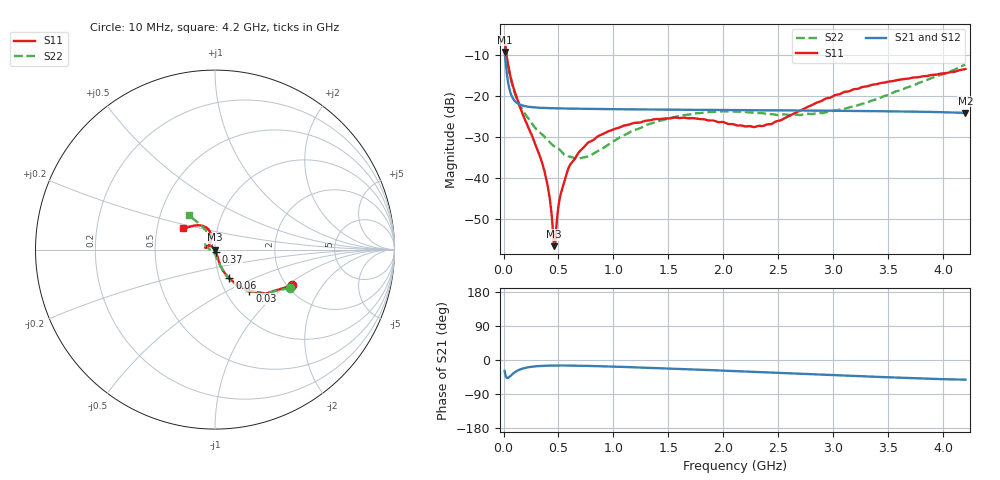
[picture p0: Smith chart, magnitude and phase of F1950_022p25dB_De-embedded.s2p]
! Integrated Device Technology
! Corporate Headquarters
! 6024 Silver Creek Valley Road
! San Jose, CA 95138  USA
! Phone:  1-408-284-8200
! Toll Free:  1-800-223-1366
! Webpage:  http://www.idt.com/
! Timing and RF Division
! 515 Groton Road, Suite 102
! Westford, MA 01886-6024
! Device:  F1950
! Description: 7-bit 0.25 dB Digital Step Attenuator
! Frequency:  150.0 -  4000.00 MHz
! Package:  4x4 mm Thin QFN Plastic Package: 24 pin
! Ports:  2 RF, 12 DC
!  Pin  1  = D0
!  Pin  2  = VDD
!  Pin  3  = Vmode
!  Pin  4  = GND
!  Pin  5  = RF1  =  Port 1
!  Pin  6  = GND
!  Pin  7  = GND
!  Pin  8  = GND
!  Pin  9  = GND
!  Pin 10  = GND
!  Pin 11  = GND
!  Pin 12  = GND
!  Pin 13  = GND
!  Pin 14  = RF2  =  Port 2
!  Pin 15  = GND
!  Pin 16  = LE
!  Pin 17  = CLK
!  Pin 18  = DATE
!  Pin 19  = D6
!  Pin 20  = D5
!  Pin 21  = D4
!  Pin 22  = D3
!  Pin 23  = D2
!  Pin 24  = D1
! State:  89
! Atten State:  22.25 dB
! Voltage:  +5.00 Volts
! Current:  Not Measured mA
! Data:  The device was measured on a the F195X evaluation board which has
!  individual transmission lines to the RF pins.  Data was collected
!  using a calibrated network analyzer.  The evaluation board was
!  de-embedded using a TRL calibration technique.
!  The reference plane is the edge of the package pin.
! Misc:  Board 2019
!  Action Tracker AT0250
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# GHz S dB R 50
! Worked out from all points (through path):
!   420 points, 10 MHz to 4.2 GHz, reference 50 ohm
!   highest |S21| = -9.31 dB at 10 MHz (marker M1); lowest = -24.1 dB at 4.2 GHz (marker M2)
!   group delay of S21, straight-line fit = 24.8 ps
!   lowest |S11| = -56.6 dB at 460 MHz (marker M3), VSWR 1.00, Z = 49.9 - j0.107 ohm
!   |S11| at or under -10 dB: 27.45 MHz to end of sweep
!   |S22| runs from -35.4 to -6.6 dB; largest |S21 - S12| = 0.00011
!   S11 on the Smith chart (normalised r, x): 10 MHz: 2.12, -1.09; 30 MHz: 1.29, -0.65; 60 MHz: 1.11, -0.37; 370 MHz: 1.01, -0.02; 4.2 GHz: 0.68, +0.17
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0.01  -6.52 -25.0  -9.31 -28.9  -9.31 -28.9  -6.61 -27.1
0.03  -10.49 -50.1  -14.54 -47.4  -14.54 -47.4  -10.80 -52.4
0.06  -14.94 -63.3  -18.95 -42.9  -18.95 -42.9  -15.12 -64.8
0.1  -18.82 -70.1  -21.16 -32.8  -21.16 -32.8  -19.17 -70.0
0.16  -23.48 -72.0  -22.24 -23.9  -22.24 -23.9  -22.86 -74.8
0.31  -33.26 -71.1  -22.87 -16.3  -22.87 -16.3  -28.42 -82.0
0.37  -38.06 -68.6  -22.95 -15.3  -22.95 -15.3  -29.87 -84.6
0.41  -43.20 -75.1  -22.99 -14.9  -22.99 -14.9  -31.01 -86.5
0.45  -52.95 -101.7  -23.02 -14.6  -23.02 -14.6  -32.05 -92.1
0.46  -56.58 -133.7  -23.03 -14.6  -23.03 -14.6  -32.25 -93.8
0.48  -52.00 155.4  -23.04 -14.5  -23.04 -14.5  -32.55 -96.7
0.52  -43.94 140.0  -23.06 -14.5  -23.06 -14.5  -33.35 -100.2
0.58  -38.41 135.0  -23.09 -14.6  -23.09 -14.6  -34.74 -112.7
0.71  -33.03 138.0  -23.14 -15.2  -23.14 -15.2  -35.09 -138.6
0.95  -28.70 146.4  -23.22 -17.0  -23.22 -17.0  -31.92 -176.3
1.41  -25.65 163.4  -23.34 -21.5  -23.35 -21.5  -26.13 160.8
1.73  -25.43 168.9  -23.40 -24.9  -23.40 -24.9  -24.30 152.4
2.11  -27.10 158.7  -23.47 -29.4  -23.47 -29.4  -23.86 142.7
2.43  -26.89 126.9  -23.52 -33.0  -23.52 -33.0  -24.43 132.0
2.81  -22.19 105.6  -23.59 -37.7  -23.58 -37.7  -24.40 116.7
3.51  -16.50 117.7  -23.75 -45.8  -23.75 -45.9  -19.69 113.5
4.2  -13.48 146.1  -24.15 -51.8  -24.14 -51.9  -12.41 127.1
